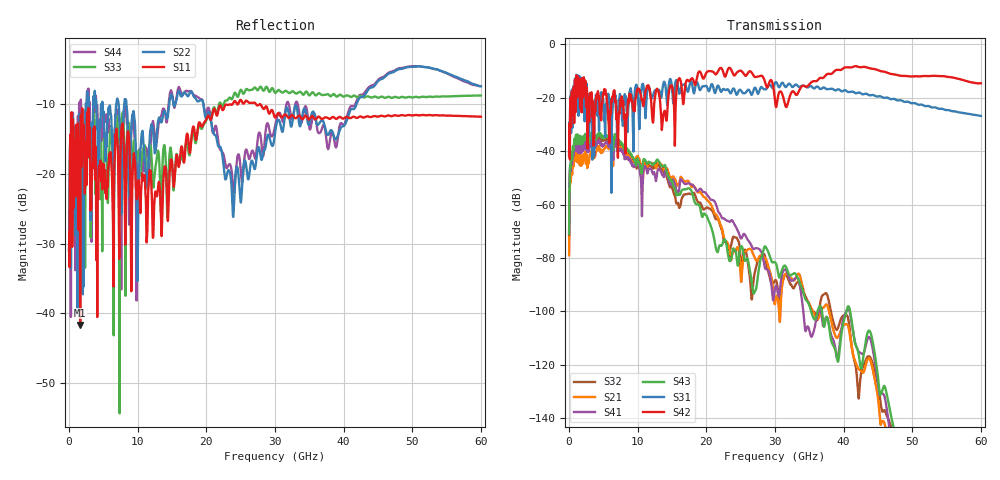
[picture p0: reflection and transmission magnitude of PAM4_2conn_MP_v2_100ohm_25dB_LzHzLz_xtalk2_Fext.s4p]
! Info: Touchstone file created by Circ.  Input file=FAB50GbE_2conn_Midplane_Examax_Topo2_v2_100ohm_25dB_LzHzLz.circ
# Hz S RI R 50
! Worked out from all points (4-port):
!   6000 points, 10 MHz to 60 GHz, reference 50 ohm
!   strongest paths, dB at 10 MHz, 15.01 GHz, 30.01 GHz, 45.01 GHz, 60 GHz:
!     S42: -41.8, -15.8, -21.2, -9.7, -14.6
!     S31: -41.3, -16.7, -14.4, -19.5, -26.8
!     S43: -71.2, -51.2, -81.6, -124.6, -171.9
!     S41: -70.5, -51.3, -91.2, -127.2, -182.4
!     S21: -79.0, -49.7, -97.1, -132.5, -177.7
!     S32: -72.9, -53.5, -88.4, -127.1, -173.9
!   lowest |S11| = -41.6 dB at 1.62 GHz (marker M1), VSWR 1.02, Z = 49.4 + j0.564 ohm
!   |S11| at or under -10 dB: start of sweep to 23.38 GHz; 27.25 GHz to 27.7 GHz (444 MHz wide, 1.62 % of centre); 27.9 GHz to end of sweep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
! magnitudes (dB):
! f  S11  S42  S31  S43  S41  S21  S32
! 10 MHz  -31.0  -41.8  -41.3  -71.2  -70.5  -79.0  -72.9
! 560 MHz  -12.2  -21.6  -20.1  -38.1  -40.8  -44.1  -39.6
! 1.62 GHz  -41.6  -23.1  -17.4  -35.1  -38.0  -41.7  -36.7
! 13.27 GHz  -22.6  -21.6  -18.4  -44.8  -47.1  -44.5  -46.3
! 23.43 GHz  -10.0  -8.9  -18.2  -81.2  -66.5  -78.2  -76.9
! 31.65 GHz  -11.6  -23.5  -15.9  -83.6  -84.7  -85.8  -86.6
! 60 GHz  -11.8  -14.6  -26.8  -171.9  -182.4  -177.7  -173.9
